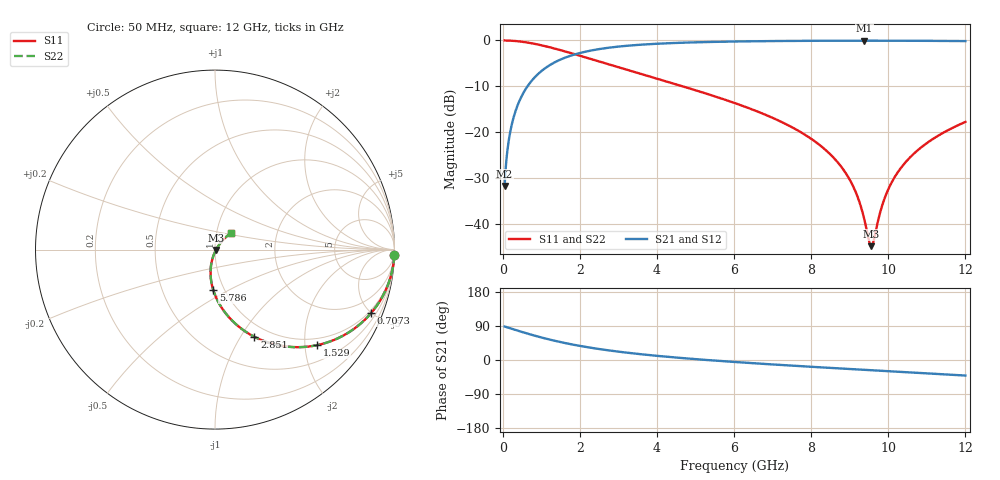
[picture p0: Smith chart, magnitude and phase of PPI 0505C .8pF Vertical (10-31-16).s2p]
# GHz S MA R 50
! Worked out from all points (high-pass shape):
!   1601 points, 50 MHz to 12 GHz, reference 50 ohm
!   highest |S21| = -0.05 dB at 9.378 GHz (marker M1); lowest = -31.8 dB at 50 MHz (marker M2)
!   |S21| within 3 dB of the highest: 1.866 GHz to end of sweep
!   lowest |S11| = -44.9 dB at 9.558 GHz (marker M3), VSWR 1.01, Z = 50.5 - j0.281 ohm
!   |S11| at or under -10 dB: 4.665 GHz to end of sweep
!   |S22| runs from -44.9 to 0.0 dB; largest |S21 - S12| = 0
!   S11 on the Smith chart (normalised r, x): 50 MHz: 1, -71; 707.2 MHz: 0.83, -4.96; 1.529 GHz: 0.84, -2.26; 2.851 GHz: 0.85, -1.15; 5.786 GHz: 0.89, -0.42; 12 GHz: 1.18, +0.22
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0.05  0.9997 -1.6  0.02582 88.4  0.02582 88.4  0.9997 -1.6
0.1620312  0.9965 -5.3  0.08344 84.7  0.08344 84.7  0.9965 -5.3
0.2815313  0.9895 -9.1  0.144 80.9  0.144 80.9  0.9895 -9.1
0.4607812  0.9726 -14.7  0.2319 75.2  0.2319 75.2  0.9726 -14.7
0.70725  0.9385 -22.2  0.3444 67.8  0.3444 67.8  0.9385 -22.2
1.528812  0.7779 -43.2  0.6266 46.7  0.6266 46.7  0.7779 -43.2
2.044156  0.6734 -53.4  0.737 36.4  0.737 36.4  0.6734 -53.4
2.850781  0.533 -65.7  0.8433 24.0  0.8433 24.0  0.533 -65.7
4.038312  0.379 -78.8  0.9219 10.7  0.9219 10.7  0.379 -78.8
5.786  0.2243 -92.6  0.9701 -3.6  0.9701 -3.6  0.2243 -92.6
6.025  0.2072 -94.1  0.9737 -5.3  0.9737 -5.3  0.2072 -94.1
8.019156  0.08363 -104.6  0.991 -18.0  0.991 -18.0  0.08363 -104.6
8.893  0.03598 -104.5  0.9934 -23.2  0.9934 -23.2  0.03598 -104.5
9.169344  0.02152 -99.9  0.9937 -24.8  0.9937 -24.8  0.02152 -99.9
9.378469  0.01121 -85.8  0.9937 -26.0  0.9937 -26.0  0.01121 -85.8
9.557719  0.005714 -29.1  0.9937 -27.0  0.9937 -27.0  0.005714 -29.1
9.624937  0.006639 2.7  0.9936 -27.4  0.9936 -27.4  0.006639 2.7
9.849  0.01623 40.2  0.9934 -28.7  0.9934 -28.7  0.01623 40.2
10.01331  0.0245 46.4  0.9932 -29.6  0.9932 -29.6  0.0245 46.4
10.327  0.04071 50.0  0.9925 -31.4  0.9925 -31.4  0.04071 50.0
10.75272  0.06296 50.4  0.9911 -33.9  0.9911 -33.9  0.06296 50.4
12  0.1293 45.9  0.984 -41.0  0.984 -41.0  0.1293 45.9
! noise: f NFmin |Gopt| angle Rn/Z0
0.05  0.001326  0.975  1.346  0.01203
1.372  0.005841  0.7724  6.724  0.005219
2.701  0.009158  0.7176  9.957  0.006365
4.031  0.0121  0.6858  13.3  0.007379
5.36  0.01488  0.6646  16.66  0.008332
6.682  0.01758  0.6501  19.98  0.009273
8.012  0.0203  0.6404  23.27  0.01025
9.341  0.02308  0.6346  26.51  0.01129
10.67  0.02596  0.6321  29.68  0.01244
12  0.02901  0.6326  32.8  0.01372
